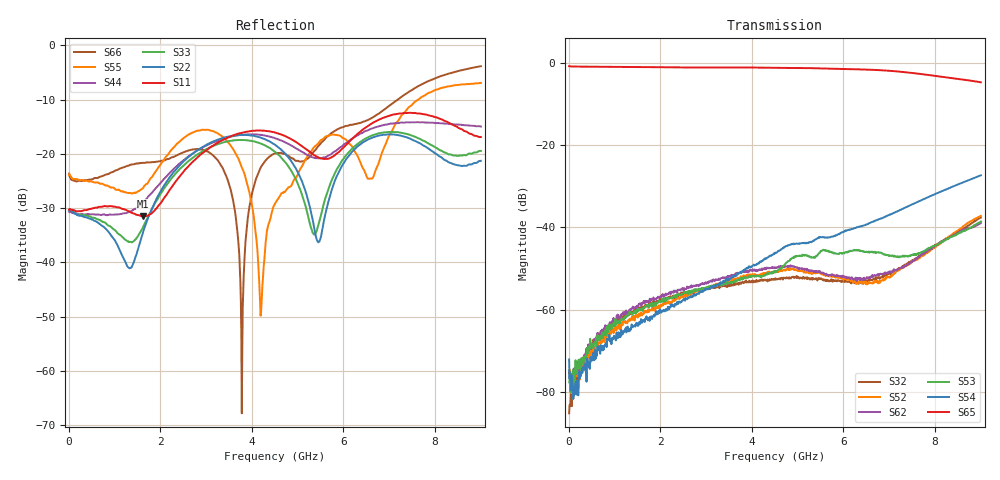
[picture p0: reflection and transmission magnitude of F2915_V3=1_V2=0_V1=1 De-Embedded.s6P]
! Integrated Device Technology
! Corporate Headquarters
! 6024 Silver Creek Valley Road
! San Jose, CA 95138  USA
! Phone:  1-408-284-8200
! Toll Free:  1-800-223-1366
! Webpage:  http://www.idt.com/
! Timing and RF Division
! 515 Groton Road, Suite 102
! Westford, MA 01886-6024
! Device:  F2915
! Description: High Reliability SP5T RF Switch
! Frequency:  0.05 -  8.GHz
! Package:  4x4 mm Thin QFN Plastic Package: 24 pin
! Ports:  6 RF,  5 DC
!  Pin  1  = GND
!  Pin  2  = RF5  =  Port 5
!  Pin  3  = GND
!  Pin  4  = GND
!  Pin  5  = RF4  =  Port 4
!  Pin  6  = GND
!  Pin  7  = GND
!  Pin  8  = RF3  =  Port 3
!  Pin  9  = GND
!  Pin 10  = GND
!  Pin 11  = RF2  =  Port 2
!  Pin 12  = GND
!  Pin 13  = GND
!  Pin 14  = RF1  =  Port 1
!  Pin 15  = GND
!  Pin 16  = Vcc
!  Pin 17  = V1
!  Pin 18  = V2
!  Pin 19  = V3
!  Pin 20  = VSSext
!  Pin 21  = GND
!  Pin 22  = RFC  =  Port 6
!  Pin 23  = GND
!  Pin 24  = GND
! Voltage:  VDD  =  +3.30 Volts
!  VSSEXT =  0.00 Volts
! Current:  IDD  = 275  uA
! State:  RF5 Selected
! V1:  Logic HIGH
! V2:  Logic LOW
! V3:  Logic HIGH
! Data:  The device was measured on the F291x evaluation board which has
!  individual transmission lines to the RF pins.  Data was collected
!  using a calibrated network analyzer.  The input lines were
!  modeled using Automatic Fixture Removal (AFR) from Keysight.
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# Hz S  dB  R 50
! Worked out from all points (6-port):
!   900 points, 10 MHz to 9 GHz, reference 50 ohm
!   strongest paths, dB at 10 MHz, 2.26 GHz, 4.51 GHz, 6.76 GHz, 9 GHz:
!     S65: -0.8, -1.1, -1.2, -1.7, -4.7
!     S54: -72.1, -59.0, -46.2, -38.1, -27.3
!     S53: -74.7, -57.2, -50.7, -46.1, -38.6
!     S62: -74.9, -55.6, -49.7, -51.5, -38.9
!     S52: -75.5, -58.3, -50.6, -53.6, -37.2
!     S32: -85.2, -56.8, -52.4, -52.1, -37.6
!   lowest |S11| = -31.5 dB at 1.62 GHz (marker M1), VSWR 1.05, Z = 49.5 + j2.6 ohm
!   |S11| at or under -10 dB: start of sweep to end of sweep
